(* Logix 5000 AddOnInstructionDefinition export Banner_T30RKD_Param_v4; software revision 33.00 *)

TYPE Banner_IOL_Port_v4 :   // UDT that has all of the data items necessary to communicate with a specific Port on a IO-Link Master
STRUCT
   Port_Controlled : INT;   // Each bit represents a port on an IO-Link Master. Set to 1 to tell AOI to control that port.
   Port_Activate : INT;   // Each bit represents a port on an IO-Link Master. When ON that port will process any commands in queue.
   Port_Read : INT;   // Each bit represents a port on an IO-Link Master. Used to determine when device AOI has requested a Read command.
   Port_Write : INT;   // Each bit represents a port on an IO-Link Master. Used to determine when device AOI has requested a Write command.
   Port_RW_Complete : INT;   // Each bit represents a port on an IO-Link Master. Tells device AOI that Read or Write request has been completed.
   Port_Device_Read : INT;
   Data_Transfer : SINT[190];   // Array to transfer data from IO-Master to device AOIs.
END_STRUCT
END_TYPE

TYPE Banner_T30RKD_RD_v4 :   // UDT that stores the Read Data for a T30RKD.
STRUCT
   Master_Cycle_Time : INT;
   Min_Cycle_Time : INT;
   M_Sequence_Capability : INT;
   IO_Link_Version_ID : INT;
   Process_Data_Input_Length : INT;
   Process_Data_Output_Length : INT;
   Combined_Vendor_ID : DINT;   // IO-Link Vendor ID
   Vendor_ID1 : INT;
   Vendor_ID2 : INT;
   Combined_Device_ID : DINT;   // IO-Link Device ID
   Device_ID1 : INT;
   Device_ID2 : INT;
   Device_ID3 : INT;
   Serial_Number : STRING;
   Teach_State : SINT;   // 0 = Idle, 1 = SP1 Success, 2 = SP2 Success, 3 = SP1 SP2 Success, 4 = Wait for command, 5 = Busy, 7 = Error
   SP1_TP1 : SINT;
   SP1_TP2 : SINT;
   SP2_TP1 : SINT;
   SP2_TP2 : SINT;
   Distance_Meaurement : DINT;
   Excess_Gain : DINT;   // Amount of singal measured over the minimum threshold.
   Stability : SINT;   // 0 = No target, 1 = Marginal target, 2 = Strong target.
   Fault_Status : SINT;   // 0 = No Fault, 1 = Fault Present
   Temperature : DINT;   // Internal Temperature.
   Last_Taught_Temperature : DINT;   // Internal Temperature the last time device was taught.
   All_Time_Run_Time : DINT;   // Read only counter that tracks the total time sensor has been running since manufacture. Value in Hours.
   MDC_Lower_Limit : DINT;
   MDC_Upper_Limit : DINT;
   MDC_Unit : INT;
   MDC_Scale : SINT;
END_STRUCT
END_TYPE

TYPE Banner_T30RKD_v4 :   // All of the parameters for a T30RKD.
STRUCT
   Initial_Global_Read : BOOL;   // Determines if all of the IO-Link data has been read into the PLC yet
   Command : INT;   // Value placed in here will activate a read or write to a specifc IO-Link Index
   Read_Data : Banner_T30RKD_RD_v4;   // Read Only Data
   Write_Data : Banner_T30RKD_WD_v4;   // Write Data
   Archive : Banner_T30RKD_WD_v4;   // Archive Data
   Reset : BOOL;   // Resets AOI. This will force a complete parameter read of the sensor.
END_STRUCT
END_TYPE

TYPE Banner_T30RKD_WD_v4 :   // UDT that stores the Write Data for a T30RKD.
STRUCT
   System_Command : INT;   // See IODD file for list of commands that can be activated via the System Command interface
   Parameter_Access_Lock : SINT;   // Write access to all parameters is prohibited while value is 1. Only this parameter can be adjusted when value is 1.
   Data_Storage_Lock : SINT;   // Automatic data storage is disabled when this value is equal to 1. Read access is not affected.
   Local_Parameterization_Lock : SINT;   // Parameterization via local control elements on device is disabled.
   Local_User_Interface_Lock : SINT;   // Operation of local user interface is disabled.
   Function_Tag : STRING;
   Location_Tag : STRING;
   Teach_in_Channel : SINT;   // 0 = Default, 1 = BDC1, 2 = BDC2
   BDC1_Setpoint_1 : DINT;   // 0 to 15000. SP1 switch point in Switch or Window mode.
   BDC1_Setpoint_2 : DINT;   // 0 to 15000. SP2 switch point in Window mode only.
   BDC1_Switchpoint_Logic : INT;   // 0 = Light Operate, 1 = Dark Operate
   BDC1_Mode : SINT;   // 1 = Switch Mode/Single Mode, 2 = Window Mode
   BDC1_Hysteresis : INT;   // 0 to 15000
   BDC2_Setpoint_1 : DINT;   // 0 to 15000. SP1 switch point in Switch or Window mode.
   BDC2_Setpoint_2 : DINT;   // 0 to 15000. SP2 switch point in Window mode only.
   BDC2_Switchpoint_Logic : INT;   // 0 = Light Operate, 1 = Dark Operate
   BDC2_Mode : SINT;   // 1 = Switch Mode/Single Mode, 2 = Window Mode
   BDC2_Hysteresis : INT;   // 0 to 15000
   Response_Speed : SINT;   // 0 = Fast, 1 = Medium, 2 = Slow
   Peak_Select_Mode : SINT;   // 0 = Strongest Peak, 1 = First Peak
   Sensor_Lockout : SINT;   // 0 = Unlocked, 1 = Locked
   Output_Polarity : SINT;   // 0 = NPN, 1 = PNP
   Process_Data_Filter_Time : INT;   // Time in ms to average process data between updates.
   Process_Data_Layout : SINT;   // 0 = Digital Measurement Sensor, 1 = Distance and Excess Gain, 2 = Distance and Excess Gain with Binary
   Remote_Input_Mode : SINT;   // 0 = Disabled, 1 = Teach
   Amplitude_Threshold : DINT;   // 100 to 5000
   Limit_Filter_Enabled : SINT;   // 0 = Disabled, 1 = Enabled. Rate of change filter for the distance meansurement.
   Limit_Filter_Hold_Time : DINT;   // 50 to 60000. Hold time for when distance change exceeds configured window.
   Limit_Filter_Positive_Distance : DINT;   // 0 to 1000. Window size for distance changes going away from sensor (set 0 to disable)
   Limit_Filter_Negative_Distance : DINT;   // 0 to 1000. Window size for distance changes going towards sensor (set 0 to disable)
   Secondary_Output_Mode : SINT;   // 0 = Independent Output, 1 = Complementary Output, 2 = Pulse Frequency Output
   BDC1_Delay_Timer_1 : DINT;   // 0 to 60000 ms.
   BDC1_Delay_Timer_2 : DINT;   // 0 to 60000 ms
   BDC1_Teach_Offset : DINT;   // -15000 to 15000. Offset applied to taught switch point during single point teach.
   BDC2_Delay_Timer_1 : DINT;   // 0 to 60000 ms
   BDC2_Delay_Timer_2 : DINT;   // 0 to 60000 ms
   BDC2_Teach_Offset : DINT;   // -15000 to 15000. Offset applied to taught switch point during single point teach.
   Resettable_Run_Time : DINT;
   Loss_of_Signal : SINT;   // 0 = Hold, 1 = Low, 2 = High
   SP1_PFM_Setpoint : DINT;   // 0 to 15000 in Hz
   SP2_PFM_Setpoint : DINT;   // 0 to 15000 in Hz
   All_Time_Run_Time_Event_Time : DINT;
   Resettable_Run_Time_Event_Time : DINT;
   Active_Sensing_Range_Near : DINT;   // 0 to 16000. Near measurement limit of sensing range.
   Active_Sensing_Range_Far : DINT;   // 0 to 16000. Far measurement limit of sensing range.
END_STRUCT
END_TYPE

ADD_ON_INSTRUCTION Banner_T30RKD_Param_v4   (* revision 4.0, vendor Banner Engineering *)
// AOI to read and write parameter data to an IO-Link T30R Dual Discrete.
VAR_IN_OUT
   T30RKD : Banner_T30RKD_v4; {required}
   Port_Data : Banner_IOL_Port_v4; {required}
END_VAR
VAR_INPUT
   Port : DINT; {required}
END_VAR
VAR
   Local_Control : DINT; {access None}
   Global_Read_Command_Value : INT; {access None}
   Global_Write_Command_Value : INT; {access None}
   Command_Being_Processed : BOOL; {access None}
   Update_Archive : BOOL; {access None}
   Index_Write_Inprocess : DINT; {access None}
   Index_Write_Control : DINT; {access None}
   Inprocess_Index : DINT; {access None}
END_VAR

ROUTINE Logic   (* ladder *)
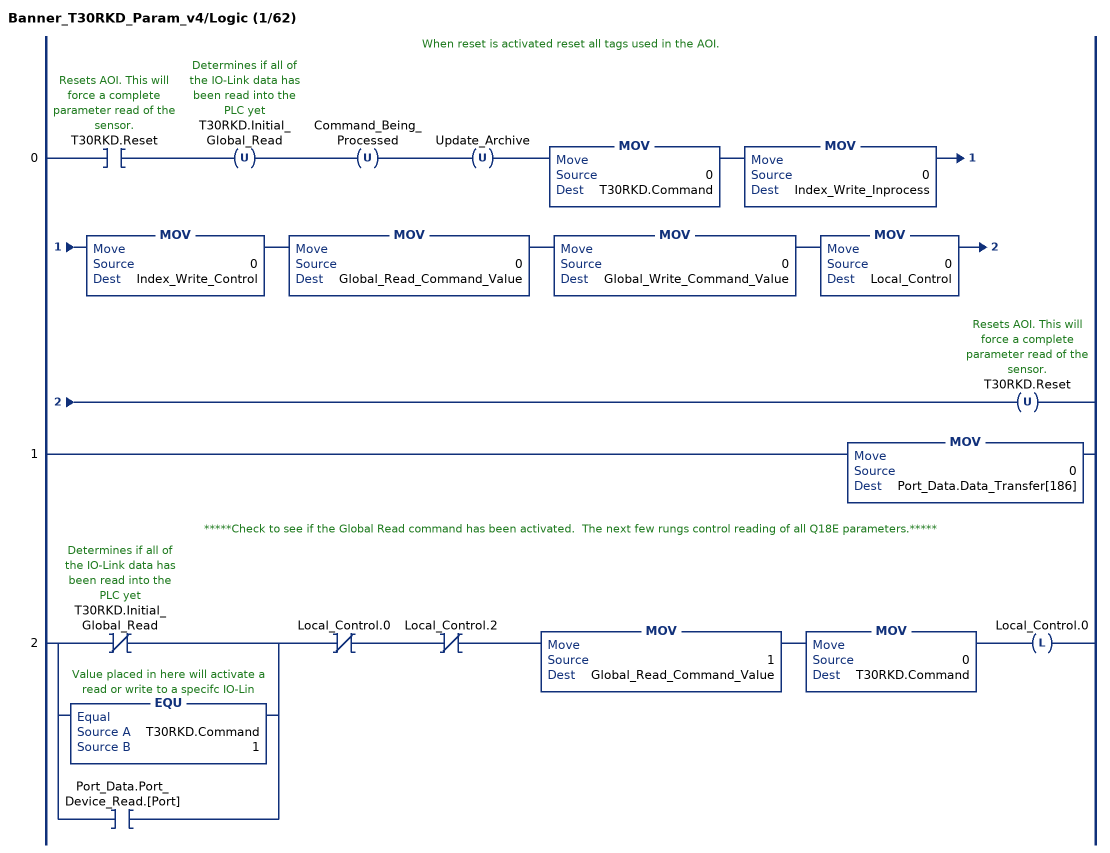
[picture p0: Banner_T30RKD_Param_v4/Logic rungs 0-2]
   // When reset is activated reset all tags used in the AOI.
   0: XIC(T30RKD.Reset)OTU(T30RKD.Initial_Global_Read)OTU(Command_Being_Processed)OTU(Update_Archive)MOV(0,T30RKD.Command)MOV(0,Index_Write_Inprocess)MOV(0,Index_Write_Control)MOV(0,Global_Read_Command_Value)MOV(0,Global_Write_Command_Value)MOV(0,Local_Control)OTU(T30RKD.Reset);
   1: MOV(0,Port_Data.Data_Transfer[186]);
   // *****Check to see if the Global Read command has been activated.  The next few rungs control reading of all Q18E parameters.*****
   2: [XIO(T30RKD.Initial_Global_Read) ,EQU(T30RKD.Command,1) ,XIC(Port_Data.Port_Device_Read.[Port]) ]XIO(Local_Control.0)XIO(Local_Control.2)MOV(1,Global_Read_Command_Value)MOV(0,T30RKD.Command)OTL(Local_Control.0);
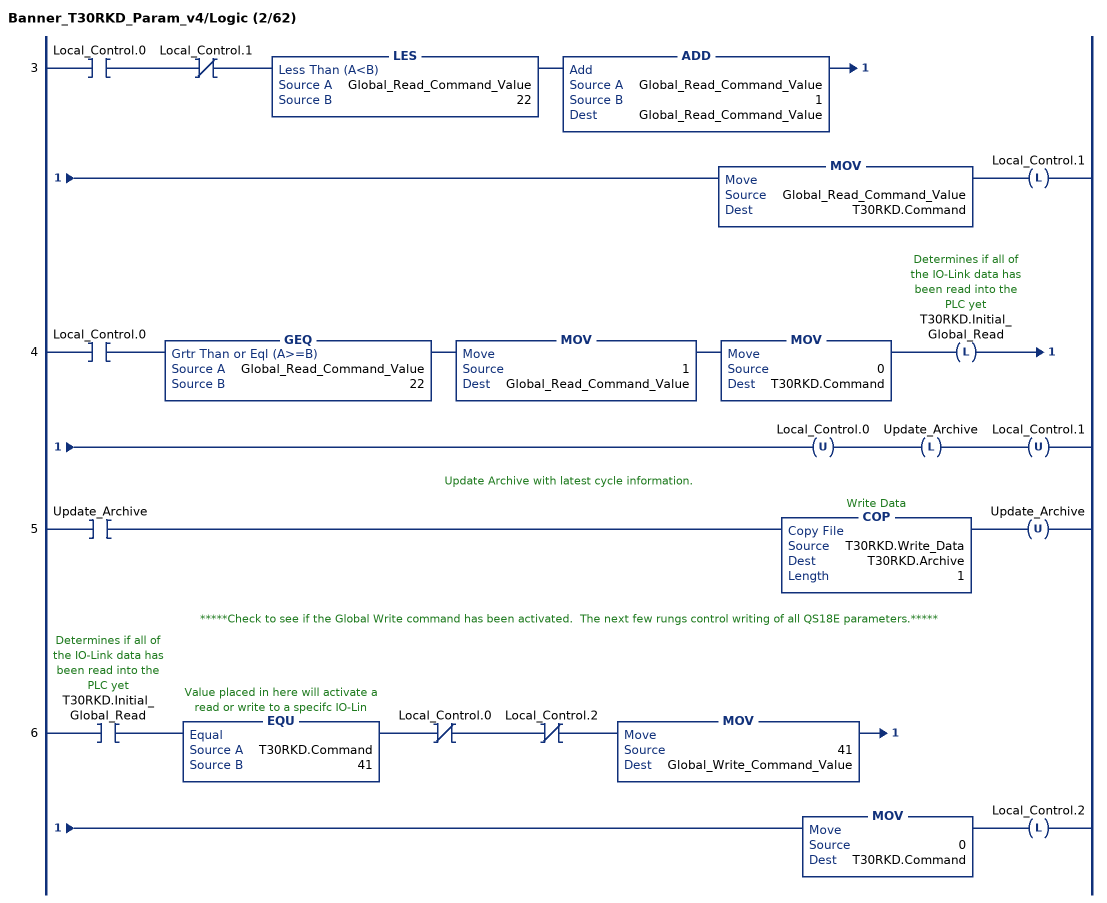
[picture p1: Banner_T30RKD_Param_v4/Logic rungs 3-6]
   3: XIC(Local_Control.0)XIO(Local_Control.1)LES(Global_Read_Command_Value,22)ADD(Global_Read_Command_Value,1,Global_Read_Command_Value)MOV(Global_Read_Command_Value,T30RKD.Command)OTL(Local_Control.1);
   4: XIC(Local_Control.0)GEQ(Global_Read_Command_Value,22)MOV(1,Global_Read_Command_Value)MOV(0,T30RKD.Command)OTL(T30RKD.Initial_Global_Read)OTU(Local_Control.0)OTL(Update_Archive)OTU(Local_Control.1);
   // Update Archive with latest cycle information.
   5: XIC(Update_Archive)COP(T30RKD.Write_Data,T30RKD.Archive,1)OTU(Update_Archive);
   // *****Check to see if the Global Write command has been activated.  The next few rungs control writing of all QS18E parameters.*****
   6: XIC(T30RKD.Initial_Global_Read)EQU(T30RKD.Command,41)XIO(Local_Control.0)XIO(Local_Control.2)MOV(41,Global_Write_Command_Value)MOV(0,T30RKD.Command)OTL(Local_Control.2);
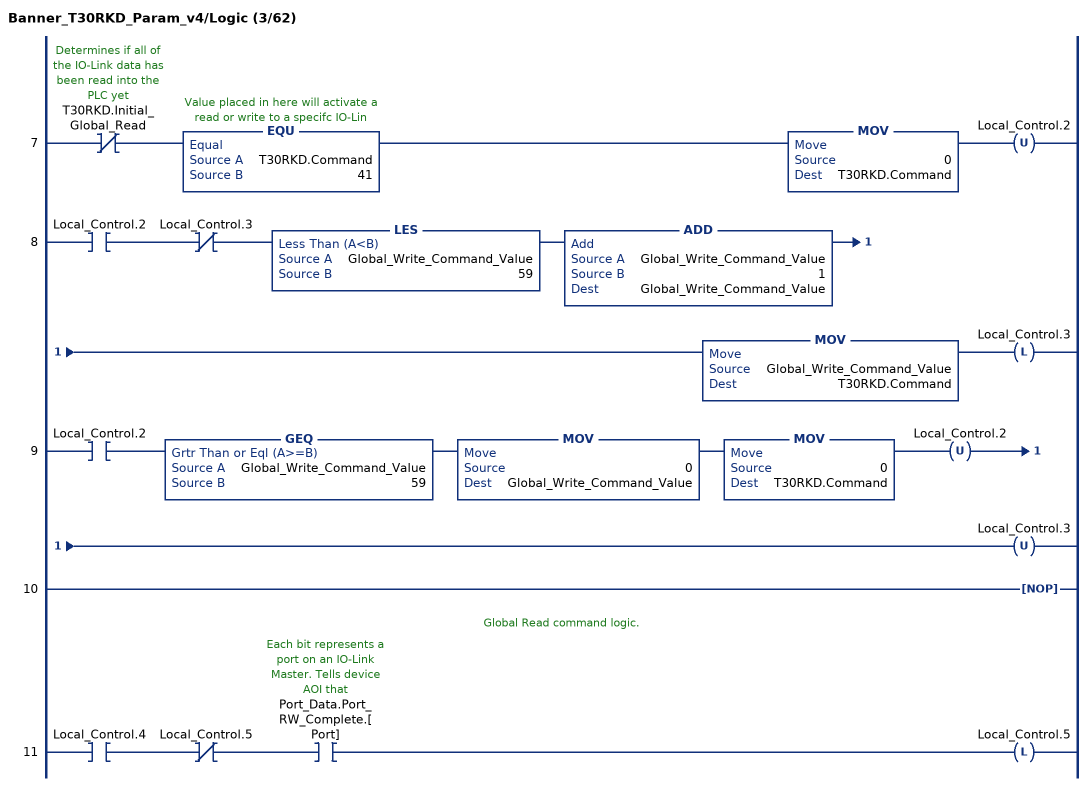
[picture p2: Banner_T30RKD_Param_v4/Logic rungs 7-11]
   7: XIO(T30RKD.Initial_Global_Read)EQU(T30RKD.Command,41)MOV(0,T30RKD.Command)OTU(Local_Control.2);
   8: XIC(Local_Control.2)XIO(Local_Control.3)LES(Global_Write_Command_Value,59)ADD(Global_Write_Command_Value,1,Global_Write_Command_Value)MOV(Global_Write_Command_Value,T30RKD.Command)OTL(Local_Control.3);
   9: XIC(Local_Control.2)GEQ(Global_Write_Command_Value,59)MOV(0,Global_Write_Command_Value)MOV(0,T30RKD.Command)OTU(Local_Control.2)OTU(Local_Control.3);
   10: NOP();
   // Global Read command logic.
   11: XIC(Local_Control.4)XIO(Local_Control.5)XIC(Port_Data.Port_RW_Complete.[Port])OTL(Local_Control.5);
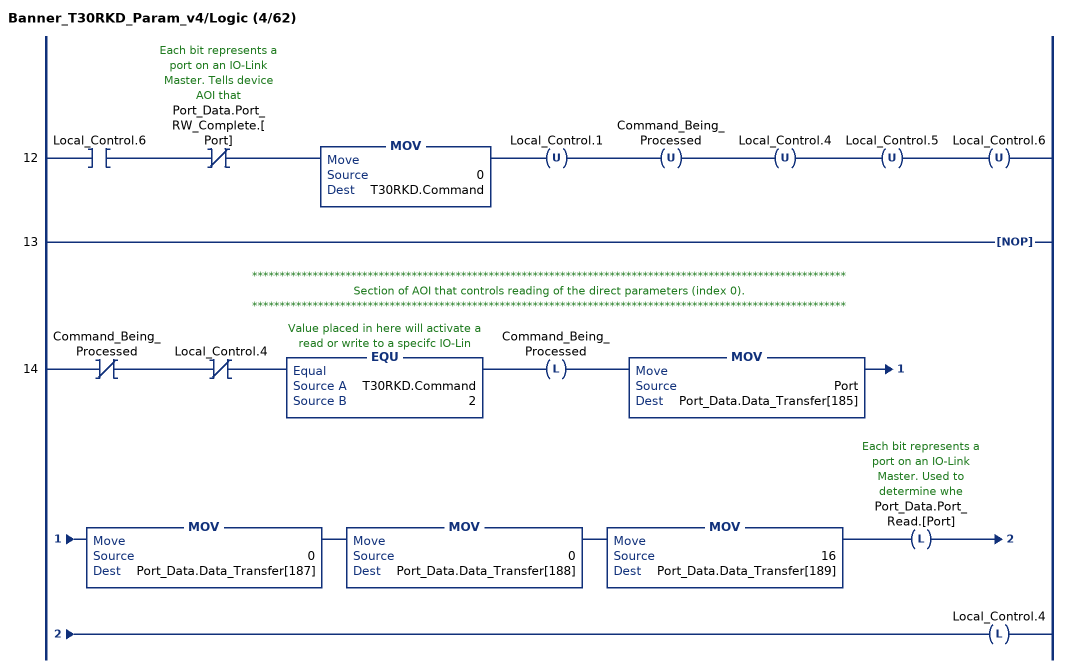
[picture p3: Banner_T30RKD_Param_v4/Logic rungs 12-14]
   12: XIC(Local_Control.6)XIO(Port_Data.Port_RW_Complete.[Port])MOV(0,T30RKD.Command)OTU(Local_Control.1)OTU(Command_Being_Processed)OTU(Local_Control.4)OTU(Local_Control.5)OTU(Local_Control.6);
   13: NOP();
   // ************************************************************************************************************
   // Section of AOI that controls reading of the direct parameters (index 0).
   // ************************************************************************************************************
   14: XIO(Command_Being_Processed)XIO(Local_Control.4)EQU(T30RKD.Command,2)OTL(Command_Being_Processed)MOV(Port,Port_Data.Data_Transfer[185])MOV(0,Port_Data.Data_Transfer[187])MOV(0,Port_Data.Data_Transfer[188])MOV(16,Port_Data.Data_Transfer[189])OTL(Port_Data.Port_Read.[Port])OTL(Local_Control.4);
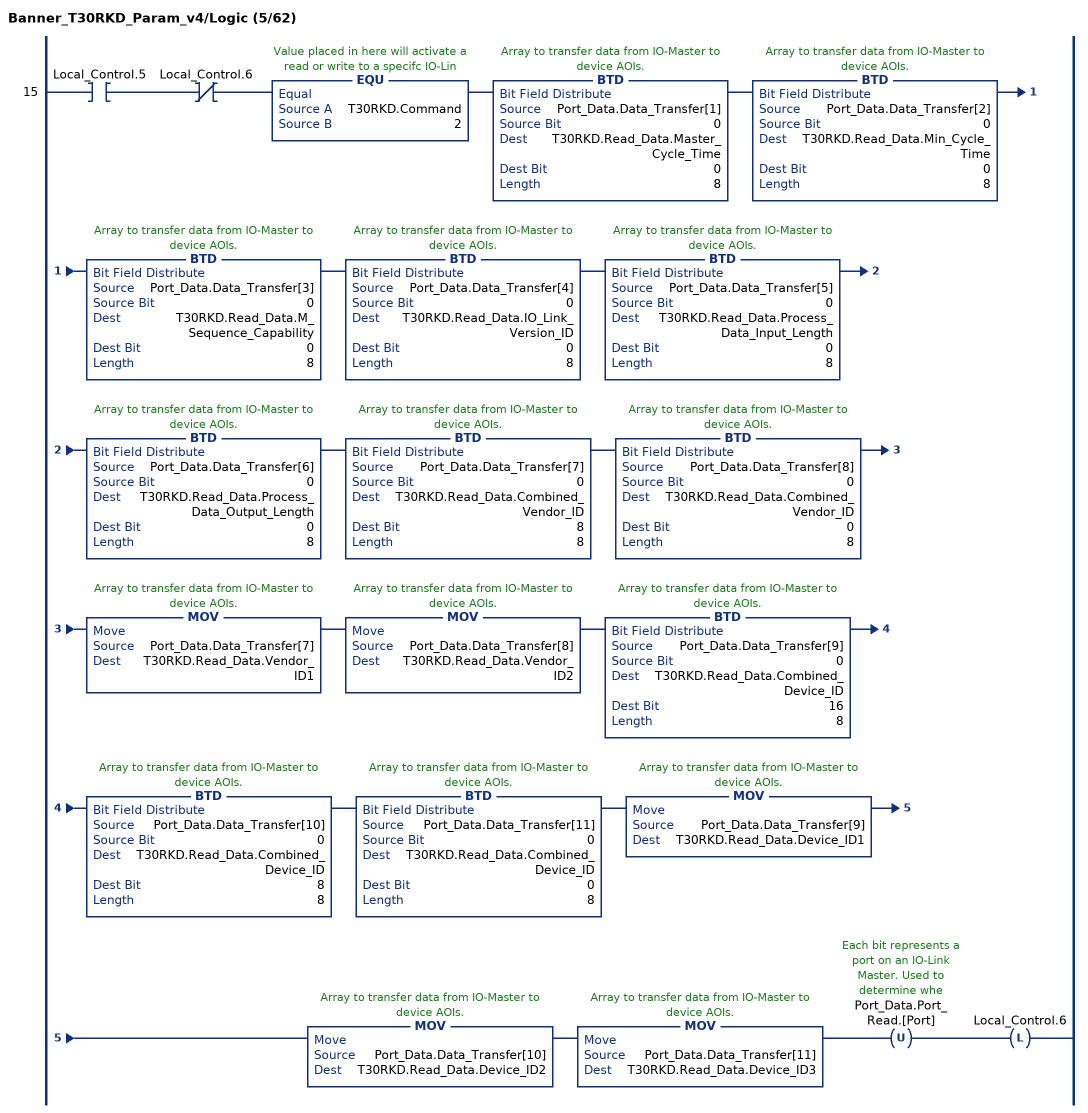
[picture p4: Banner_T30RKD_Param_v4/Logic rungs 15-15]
   15: XIC(Local_Control.5)XIO(Local_Control.6)EQU(T30RKD.Command,2)BTD(Port_Data.Data_Transfer[1],0,T30RKD.Read_Data.Master_Cycle_Time,0,8)BTD(Port_Data.Data_Transfer[2],0,T30RKD.Read_Data.Min_Cycle_Time,0,8)BTD(Port_Data.Data_Transfer[3],0,T30RKD.Read_Data.M_Sequence_Capability,0,8)BTD(Port_Data.Data_Transfer[4],0,T30RKD.Read_Data.IO_Link_Version_ID,0,8)BTD(Port_Data.Data_Transfer[5],0,T30RKD.Read_Data.Process_Data_Input_Length,0,8)BTD(Port_Data.Data_Transfer[6],0,T30RKD.Read_Data.Process_Data_Output_Length,0,8)BTD(Port_Data.Data_Transfer[7],0,T30RKD.Read_Data.Combined_Vendor_ID,8,8)BTD(Port_Data.Data_Transfer[8],0,T30RKD.Read_Data.Combined_Vendor_ID,0,8)MOV(Port_Data.Data_Transfer[7],T30RKD.Read_Data.Vendor_ID1)MOV(Port_Data.Data_Transfer[8],T30RKD.Read_Data.Vendor_ID2)BTD(Port_Data.Data_Transfer[9],0,T30RKD.Read_Data.Combined_Device_ID,16,8)BTD(Port_Data.Data_Transfer[10],0,T30RKD.Read_Data.Combined_Device_ID,8,8)BTD(Port_Data.Data_Transfer[11],0,T30RKD.Read_Data.Combined_Device_ID,0,8)MOV(Port_Data.Data_Transfer[9],T30RKD.Read_Data.Device_ID1)MOV(Port_Data.Data_Transfer[10],T30RKD.Read_Data.Device_ID2)MOV(Port_Data.Data_Transfer[11],T30RKD.Read_Data.Device_ID3)OTU(Port_Data.Port_Read.[Port])OTL(Local_Control.6);
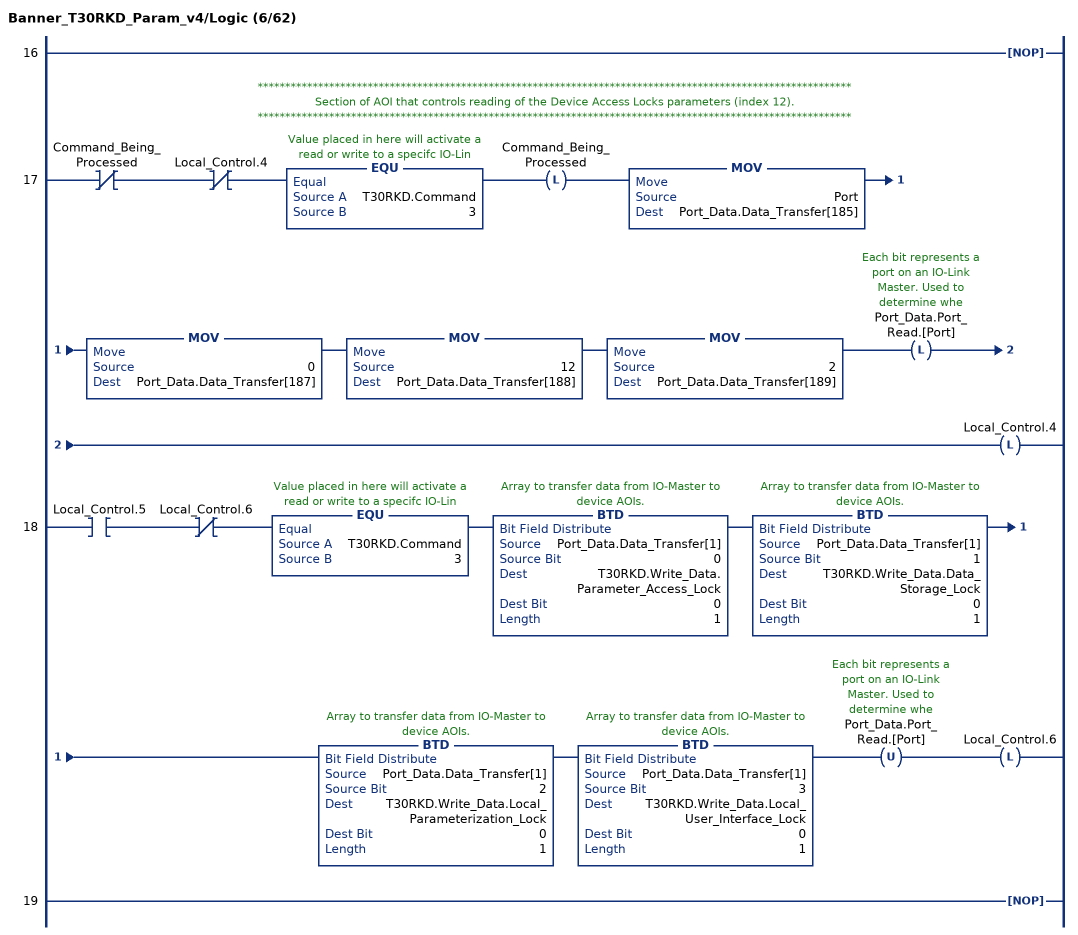
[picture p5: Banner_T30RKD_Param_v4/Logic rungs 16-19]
   16: NOP();
   // ************************************************************************************************************
   // Section of AOI that controls reading of the Device Access Locks parameters (index 12).
   // ************************************************************************************************************
   17: XIO(Command_Being_Processed)XIO(Local_Control.4)EQU(T30RKD.Command,3)OTL(Command_Being_Processed)MOV(Port,Port_Data.Data_Transfer[185])MOV(0,Port_Data.Data_Transfer[187])MOV(12,Port_Data.Data_Transfer[188])MOV(2,Port_Data.Data_Transfer[189])OTL(Port_Data.Port_Read.[Port])OTL(Local_Control.4);
   18: XIC(Local_Control.5)XIO(Local_Control.6)EQU(T30RKD.Command,3)BTD(Port_Data.Data_Transfer[1],0,T30RKD.Write_Data.Parameter_Access_Lock,0,1)BTD(Port_Data.Data_Transfer[1],1,T30RKD.Write_Data.Data_Storage_Lock,0,1)BTD(Port_Data.Data_Transfer[1],2,T30RKD.Write_Data.Local_Parameterization_Lock,0,1)BTD(Port_Data.Data_Transfer[1],3,T30RKD.Write_Data.Local_User_Interface_Lock,0,1)OTU(Port_Data.Port_Read.[Port])OTL(Local_Control.6);
   19: NOP();
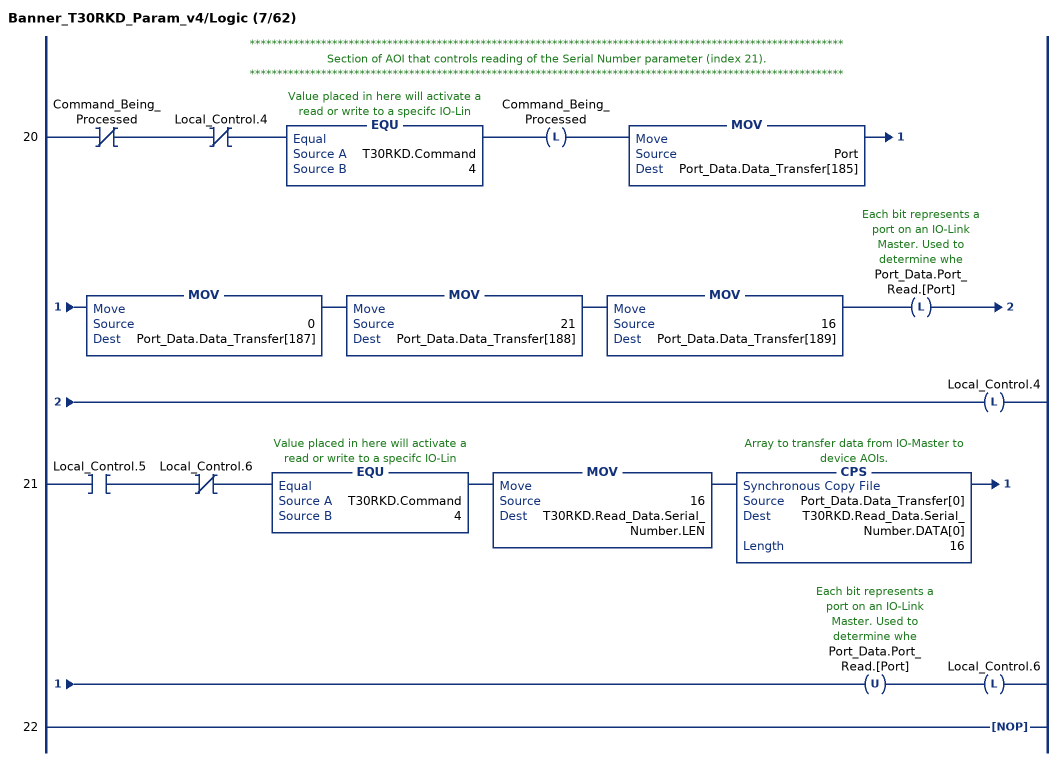
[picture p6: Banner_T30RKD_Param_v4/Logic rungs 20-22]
   // ************************************************************************************************************
   // Section of AOI that controls reading of the Serial Number parameter (index 21).
   // ************************************************************************************************************
   20: XIO(Command_Being_Processed)XIO(Local_Control.4)EQU(T30RKD.Command,4)OTL(Command_Being_Processed)MOV(Port,Port_Data.Data_Transfer[185])MOV(0,Port_Data.Data_Transfer[187])MOV(21,Port_Data.Data_Transfer[188])MOV(16,Port_Data.Data_Transfer[189])OTL(Port_Data.Port_Read.[Port])OTL(Local_Control.4);
   21: XIC(Local_Control.5)XIO(Local_Control.6)EQU(T30RKD.Command,4)MOV(16,T30RKD.Read_Data.Serial_Number.LEN)CPS(Port_Data.Data_Transfer[0],T30RKD.Read_Data.Serial_Number.DATA[0],16)OTU(Port_Data.Port_Read.[Port])OTL(Local_Control.6);
   22: NOP();
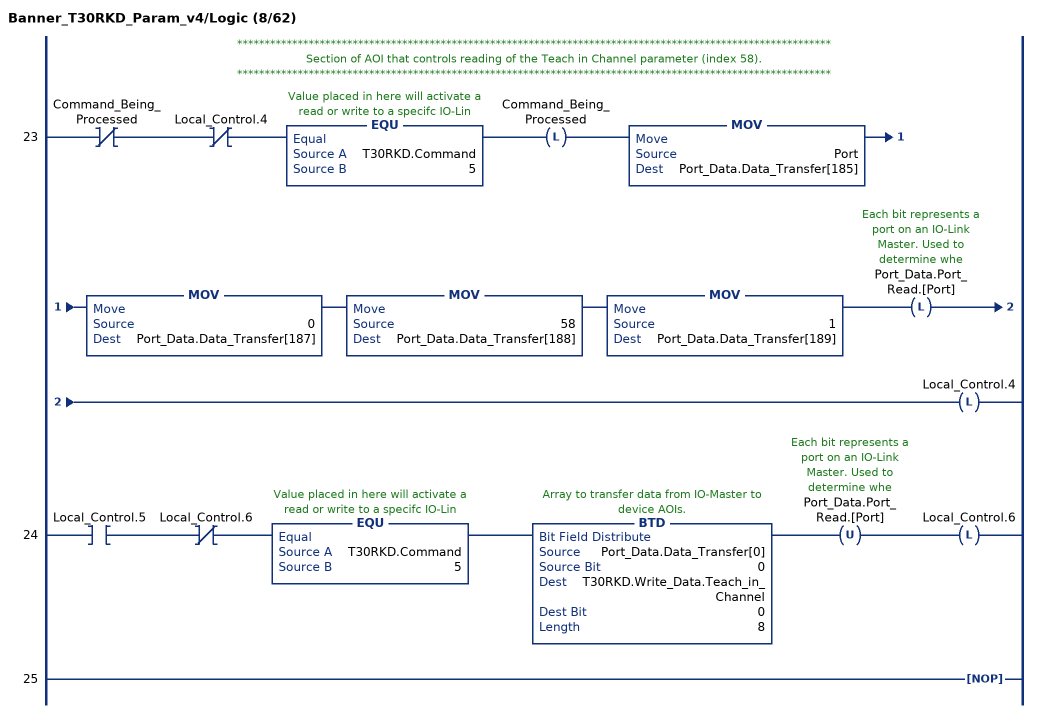
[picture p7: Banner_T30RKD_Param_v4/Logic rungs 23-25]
   // ************************************************************************************************************
   // Section of AOI that controls reading of the Teach in Channel parameter (index 58).
   // ************************************************************************************************************
   23: XIO(Command_Being_Processed)XIO(Local_Control.4)EQU(T30RKD.Command,5)OTL(Command_Being_Processed)MOV(Port,Port_Data.Data_Transfer[185])MOV(0,Port_Data.Data_Transfer[187])MOV(58,Port_Data.Data_Transfer[188])MOV(1,Port_Data.Data_Transfer[189])OTL(Port_Data.Port_Read.[Port])OTL(Local_Control.4);
   24: XIC(Local_Control.5)XIO(Local_Control.6)EQU(T30RKD.Command,5)BTD(Port_Data.Data_Transfer[0],0,T30RKD.Write_Data.Teach_in_Channel,0,8)OTU(Port_Data.Port_Read.[Port])OTL(Local_Control.6);
   25: NOP();
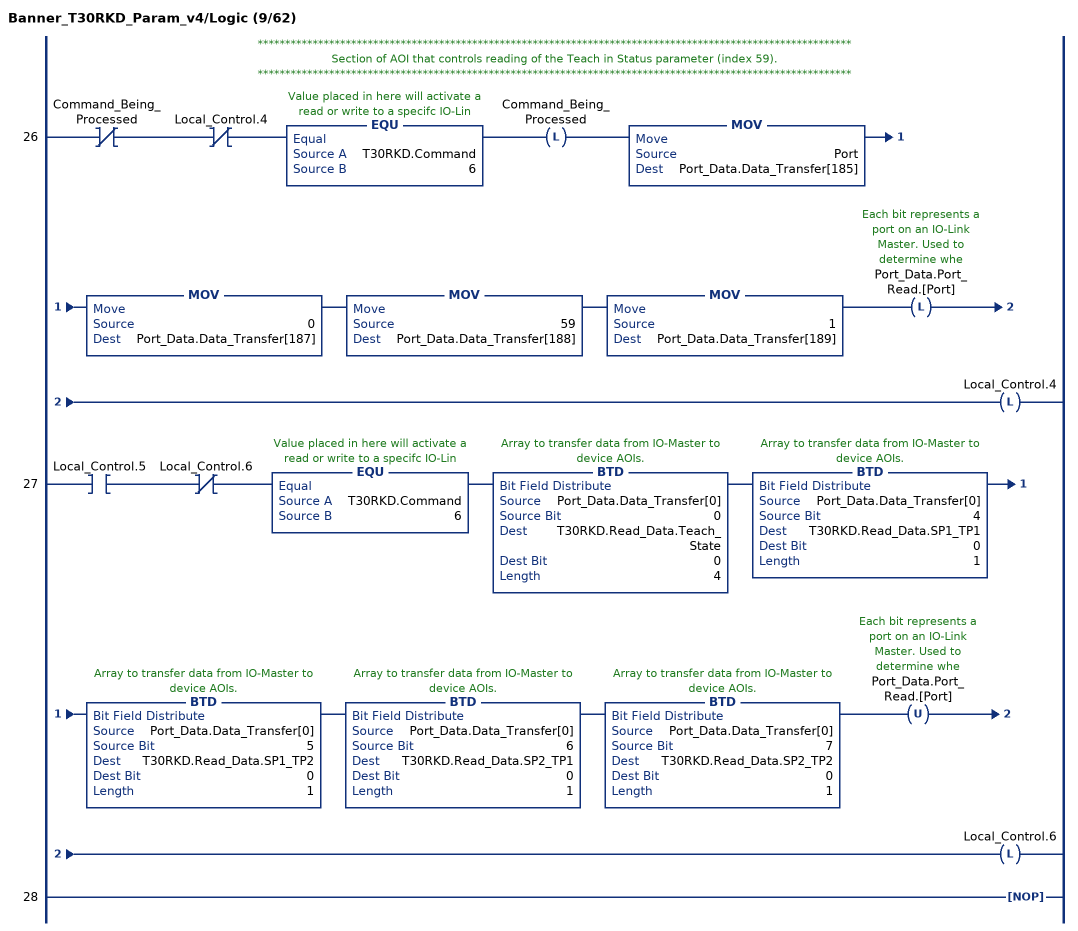
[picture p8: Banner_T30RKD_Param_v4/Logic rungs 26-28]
   // ************************************************************************************************************
   // Section of AOI that controls reading of the Teach in Status parameter (index 59).
   // ************************************************************************************************************
   26: XIO(Command_Being_Processed)XIO(Local_Control.4)EQU(T30RKD.Command,6)OTL(Command_Being_Processed)MOV(Port,Port_Data.Data_Transfer[185])MOV(0,Port_Data.Data_Transfer[187])MOV(59,Port_Data.Data_Transfer[188])MOV(1,Port_Data.Data_Transfer[189])OTL(Port_Data.Port_Read.[Port])OTL(Local_Control.4);
   27: XIC(Local_Control.5)XIO(Local_Control.6)EQU(T30RKD.Command,6)BTD(Port_Data.Data_Transfer[0],0,T30RKD.Read_Data.Teach_State,0,4)BTD(Port_Data.Data_Transfer[0],4,T30RKD.Read_Data.SP1_TP1,0,1)BTD(Port_Data.Data_Transfer[0],5,T30RKD.Read_Data.SP1_TP2,0,1)BTD(Port_Data.Data_Transfer[0],6,T30RKD.Read_Data.SP2_TP1,0,1)BTD(Port_Data.Data_Transfer[0],7,T30RKD.Read_Data.SP2_TP2,0,1)OTU(Port_Data.Port_Read.[Port])OTL(Local_Control.6);
   28: NOP();
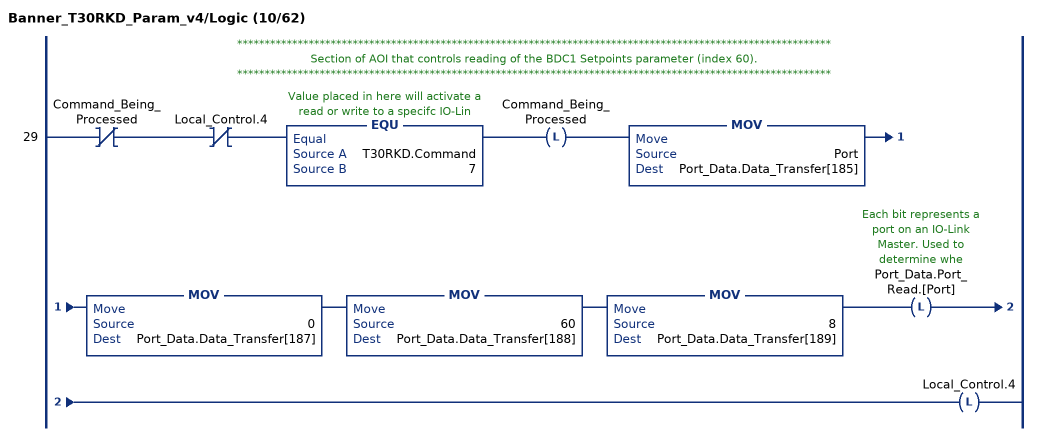
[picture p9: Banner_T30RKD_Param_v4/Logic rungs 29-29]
   // ************************************************************************************************************
   // Section of AOI that controls reading of the BDC1 Setpoints parameter (index 60).
   // ************************************************************************************************************
   29: XIO(Command_Being_Processed)XIO(Local_Control.4)EQU(T30RKD.Command,7)OTL(Command_Being_Processed)MOV(Port,Port_Data.Data_Transfer[185])MOV(0,Port_Data.Data_Transfer[187])MOV(60,Port_Data.Data_Transfer[188])MOV(8,Port_Data.Data_Transfer[189])OTL(Port_Data.Port_Read.[Port])OTL(Local_Control.4);
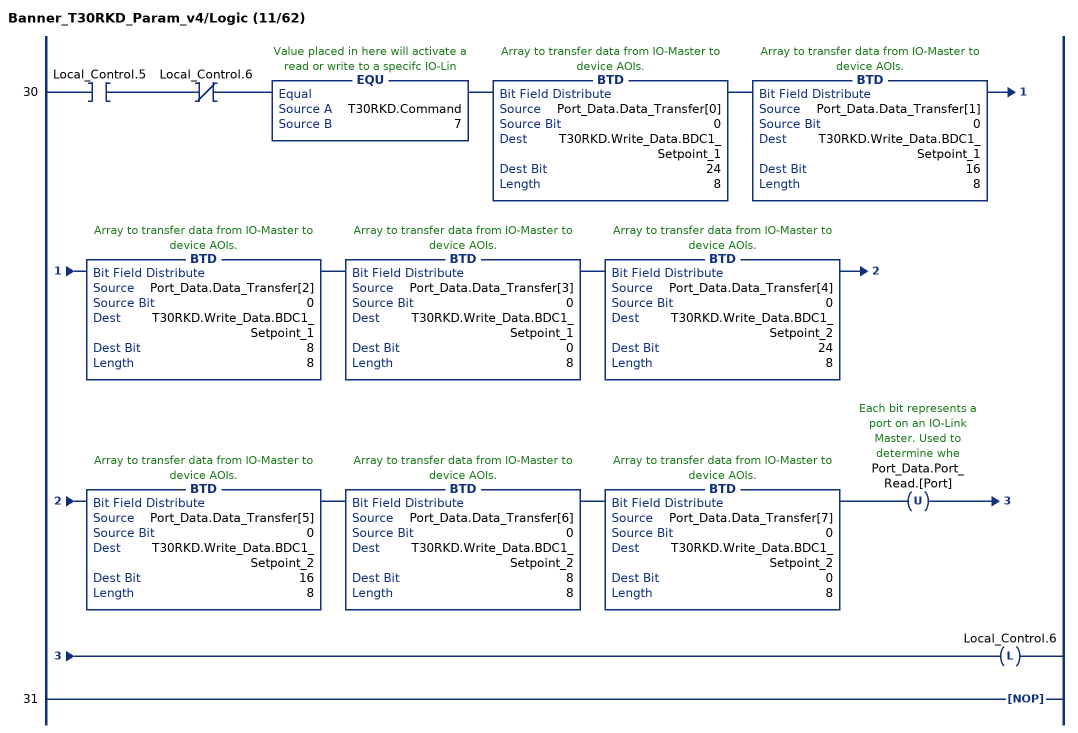
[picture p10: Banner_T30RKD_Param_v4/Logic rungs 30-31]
   30: XIC(Local_Control.5)XIO(Local_Control.6)EQU(T30RKD.Command,7)BTD(Port_Data.Data_Transfer[0],0,T30RKD.Write_Data.BDC1_Setpoint_1,24,8)BTD(Port_Data.Data_Transfer[1],0,T30RKD.Write_Data.BDC1_Setpoint_1,16,8)BTD(Port_Data.Data_Transfer[2],0,T30RKD.Write_Data.BDC1_Setpoint_1,8,8)BTD(Port_Data.Data_Transfer[3],0,T30RKD.Write_Data.BDC1_Setpoint_1,0,8)BTD(Port_Data.Data_Transfer[4],0,T30RKD.Write_Data.BDC1_Setpoint_2,24,8)BTD(Port_Data.Data_Transfer[5],0,T30RKD.Write_Data.BDC1_Setpoint_2,16,8)BTD(Port_Data.Data_Transfer[6],0,T30RKD.Write_Data.BDC1_Setpoint_2,8,8)BTD(Port_Data.Data_Transfer[7],0,T30RKD.Write_Data.BDC1_Setpoint_2,0,8)OTU(Port_Data.Port_Read.[Port])OTL(Local_Control.6);
   31: NOP();
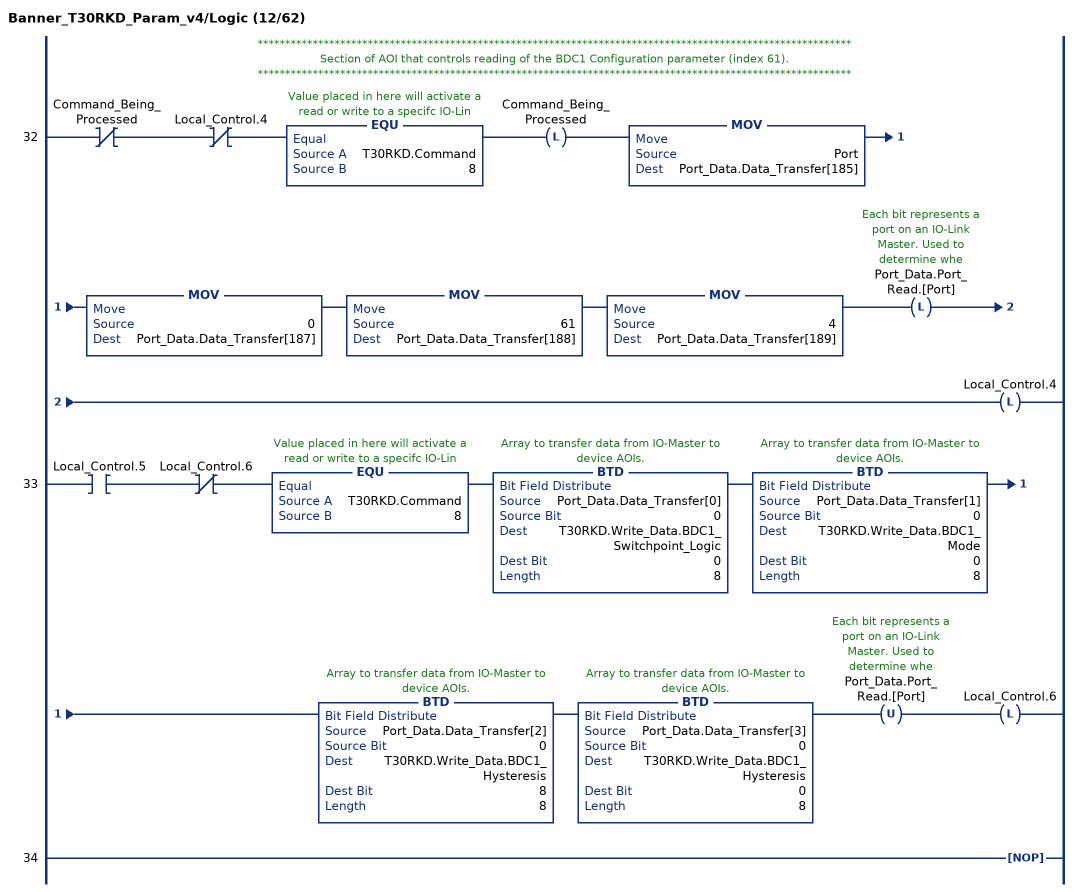
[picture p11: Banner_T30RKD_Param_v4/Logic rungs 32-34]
   // ************************************************************************************************************
   // Section of AOI that controls reading of the BDC1 Configuration parameter (index 61).
   // ************************************************************************************************************
   32: XIO(Command_Being_Processed)XIO(Local_Control.4)EQU(T30RKD.Command,8)OTL(Command_Being_Processed)MOV(Port,Port_Data.Data_Transfer[185])MOV(0,Port_Data.Data_Transfer[187])MOV(61,Port_Data.Data_Transfer[188])MOV(4,Port_Data.Data_Transfer[189])OTL(Port_Data.Port_Read.[Port])OTL(Local_Control.4);
   33: XIC(Local_Control.5)XIO(Local_Control.6)EQU(T30RKD.Command,8)BTD(Port_Data.Data_Transfer[0],0,T30RKD.Write_Data.BDC1_Switchpoint_Logic,0,8)BTD(Port_Data.Data_Transfer[1],0,T30RKD.Write_Data.BDC1_Mode,0,8)BTD(Port_Data.Data_Transfer[2],0,T30RKD.Write_Data.BDC1_Hysteresis,8,8)BTD(Port_Data.Data_Transfer[3],0,T30RKD.Write_Data.BDC1_Hysteresis,0,8)OTU(Port_Data.Port_Read.[Port])OTL(Local_Control.6);
   34: NOP();
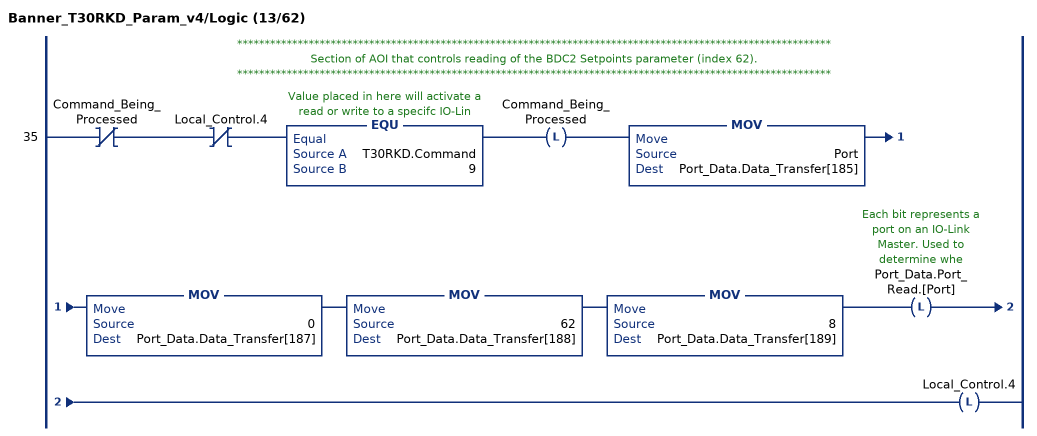
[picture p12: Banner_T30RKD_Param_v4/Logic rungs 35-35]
   // ************************************************************************************************************
   // Section of AOI that controls reading of the BDC2 Setpoints parameter (index 62).
   // ************************************************************************************************************
   35: XIO(Command_Being_Processed)XIO(Local_Control.4)EQU(T30RKD.Command,9)OTL(Command_Being_Processed)MOV(Port,Port_Data.Data_Transfer[185])MOV(0,Port_Data.Data_Transfer[187])MOV(62,Port_Data.Data_Transfer[188])MOV(8,Port_Data.Data_Transfer[189])OTL(Port_Data.Port_Read.[Port])OTL(Local_Control.4);
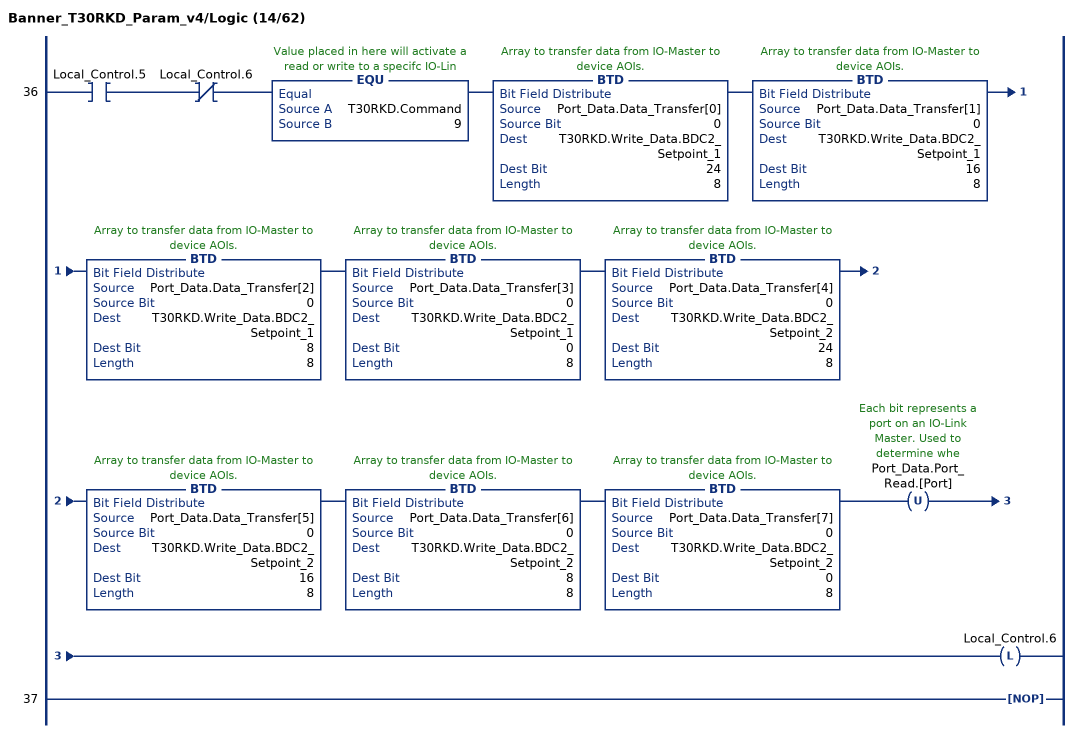
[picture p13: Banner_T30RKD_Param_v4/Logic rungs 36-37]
   36: XIC(Local_Control.5)XIO(Local_Control.6)EQU(T30RKD.Command,9)BTD(Port_Data.Data_Transfer[0],0,T30RKD.Write_Data.BDC2_Setpoint_1,24,8)BTD(Port_Data.Data_Transfer[1],0,T30RKD.Write_Data.BDC2_Setpoint_1,16,8)BTD(Port_Data.Data_Transfer[2],0,T30RKD.Write_Data.BDC2_Setpoint_1,8,8)BTD(Port_Data.Data_Transfer[3],0,T30RKD.Write_Data.BDC2_Setpoint_1,0,8)BTD(Port_Data.Data_Transfer[4],0,T30RKD.Write_Data.BDC2_Setpoint_2,24,8)BTD(Port_Data.Data_Transfer[5],0,T30RKD.Write_Data.BDC2_Setpoint_2,16,8)BTD(Port_Data.Data_Transfer[6],0,T30RKD.Write_Data.BDC2_Setpoint_2,8,8)BTD(Port_Data.Data_Transfer[7],0,T30RKD.Write_Data.BDC2_Setpoint_2,0,8)OTU(Port_Data.Port_Read.[Port])OTL(Local_Control.6);
   37: NOP();
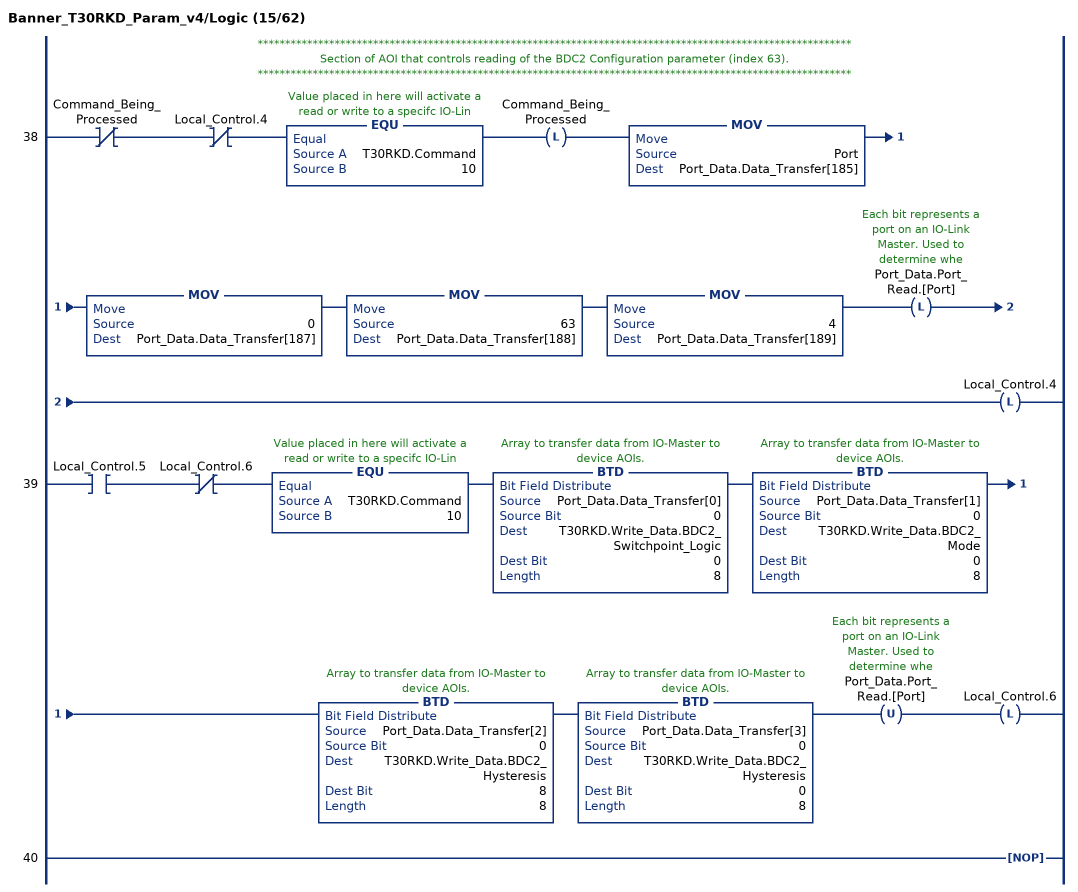
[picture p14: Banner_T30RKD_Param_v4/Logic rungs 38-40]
   // ************************************************************************************************************
   // Section of AOI that controls reading of the BDC2 Configuration parameter (index 63).
   // ************************************************************************************************************
   38: XIO(Command_Being_Processed)XIO(Local_Control.4)EQU(T30RKD.Command,10)OTL(Command_Being_Processed)MOV(Port,Port_Data.Data_Transfer[185])MOV(0,Port_Data.Data_Transfer[187])MOV(63,Port_Data.Data_Transfer[188])MOV(4,Port_Data.Data_Transfer[189])OTL(Port_Data.Port_Read.[Port])OTL(Local_Control.4);
   39: XIC(Local_Control.5)XIO(Local_Control.6)EQU(T30RKD.Command,10)BTD(Port_Data.Data_Transfer[0],0,T30RKD.Write_Data.BDC2_Switchpoint_Logic,0,8)BTD(Port_Data.Data_Transfer[1],0,T30RKD.Write_Data.BDC2_Mode,0,8)BTD(Port_Data.Data_Transfer[2],0,T30RKD.Write_Data.BDC2_Hysteresis,8,8)BTD(Port_Data.Data_Transfer[3],0,T30RKD.Write_Data.BDC2_Hysteresis,0,8)OTU(Port_Data.Port_Read.[Port])OTL(Local_Control.6);
   40: NOP();
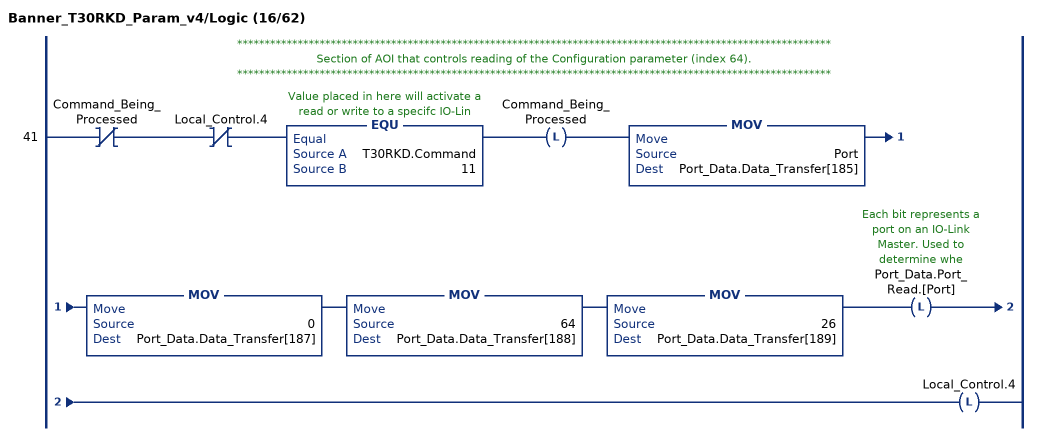
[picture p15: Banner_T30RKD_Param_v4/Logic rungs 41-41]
   // ************************************************************************************************************
   // Section of AOI that controls reading of the Configuration parameter (index 64).
   // ************************************************************************************************************
   41: XIO(Command_Being_Processed)XIO(Local_Control.4)EQU(T30RKD.Command,11)OTL(Command_Being_Processed)MOV(Port,Port_Data.Data_Transfer[185])MOV(0,Port_Data.Data_Transfer[187])MOV(64,Port_Data.Data_Transfer[188])MOV(26,Port_Data.Data_Transfer[189])OTL(Port_Data.Port_Read.[Port])OTL(Local_Control.4);
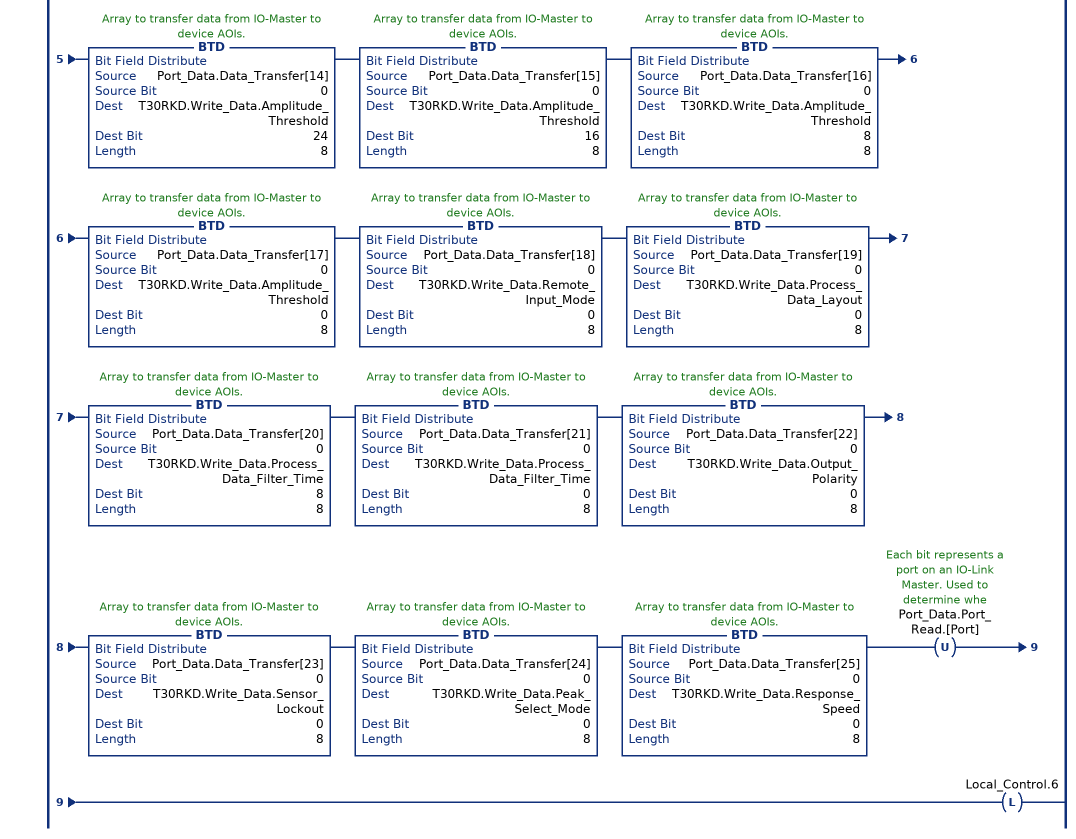
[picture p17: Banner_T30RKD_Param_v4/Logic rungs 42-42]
   42: XIC(Local_Control.5)XIO(Local_Control.6)EQU(T30RKD.Command,11)BTD(Port_Data.Data_Transfer[0],0,T30RKD.Write_Data.Secondary_Output_Mode,0,8)BTD(Port_Data.Data_Transfer[1],0,T30RKD.Write_Data.Limit_Filter_Negative_Distance,24,8)BTD(Port_Data.Data_Transfer[2],0,T30RKD.Write_Data.Limit_Filter_Negative_Distance,16,8)BTD(Port_Data.Data_Transfer[3],0,T30RKD.Write_Data.Limit_Filter_Negative_Distance,8,8)BTD(Port_Data.Data_Transfer[4],0,T30RKD.Write_Data.Limit_Filter_Negative_Distance,0,8)BTD(Port_Data.Data_Transfer[5],0,T30RKD.Write_Data.Limit_Filter_Positive_Distance,24,8)BTD(Port_Data.Data_Transfer[6],0,T30RKD.Write_Data.Limit_Filter_Positive_Distance,16,8)BTD(Port_Data.Data_Transfer[7],0,T30RKD.Write_Data.Limit_Filter_Positive_Distance,8,8)BTD(Port_Data.Data_Transfer[8],0,T30RKD.Write_Data.Limit_Filter_Positive_Distance,0,8)BTD(Port_Data.Data_Transfer[9],0,T30RKD.Write_Data.Limit_Filter_Hold_Time,24,8)BTD(Port_Data.Data_Transfer[10],0,T30RKD.Write_Data.Limit_Filter_Hold_Time,16,8)BTD(Port_Data.Data_Transfer[11],0,T30RKD.Write_Data.Limit_Filter_Hold_Time,8,8)BTD(Port_Data.Data_Transfer[12],0,T30RKD.Write_Data.Limit_Filter_Hold_Time,0,8)BTD(Port_Data.Data_Transfer[13],0,T30RKD.Write_Data.Limit_Filter_Enabled,0,8)BTD(Port_Data.Data_Transfer[14],0,T30RKD.Write_Data.Amplitude_Threshold,24,8)BTD(Port_Data.Data_Transfer[15],0,T30RKD.Write_Data.Amplitude_Threshold,16,8)BTD(Port_Data.Data_Transfer[16],0,T30RKD.Write_Data.Amplitude_Threshold,8,8)BTD(Port_Data.Data_Transfer[17],0,T30RKD.Write_Data.Amplitude_Threshold,0,8)BTD(Port_Data.Data_Transfer[18],0,T30RKD.Write_Data.Remote_Input_Mode,0,8)BTD(Port_Data.Data_Transfer[19],0,T30RKD.Write_Data.Process_Data_Layout,0,8)BTD(Port_Data.Data_Transfer[20],0,T30RKD.Write_Data.Process_Data_Filter_Time,8,8)BTD(Port_Data.Data_Transfer[21],0,T30RKD.Write_Data.Process_Data_Filter_Time,0,8)BTD(Port_Data.Data_Transfer[22],0,T30RKD.Write_Data.Output_Polarity,0,8)BTD(Port_Data.Data_Transfer[23],0,T30RKD.Write_Data.Sensor_Lockout,0,8)BTD(Port_Data.Data_Transfer[24],0,T30RKD.Write_Data.Peak_Select_Mode,0,8)BTD(Port_Data.Data_Transfer[25],0,T30RKD.Write_Data.Response_Speed,0,8)OTU(Port_Data.Port_Read.[Port])OTL(Local_Control.6);
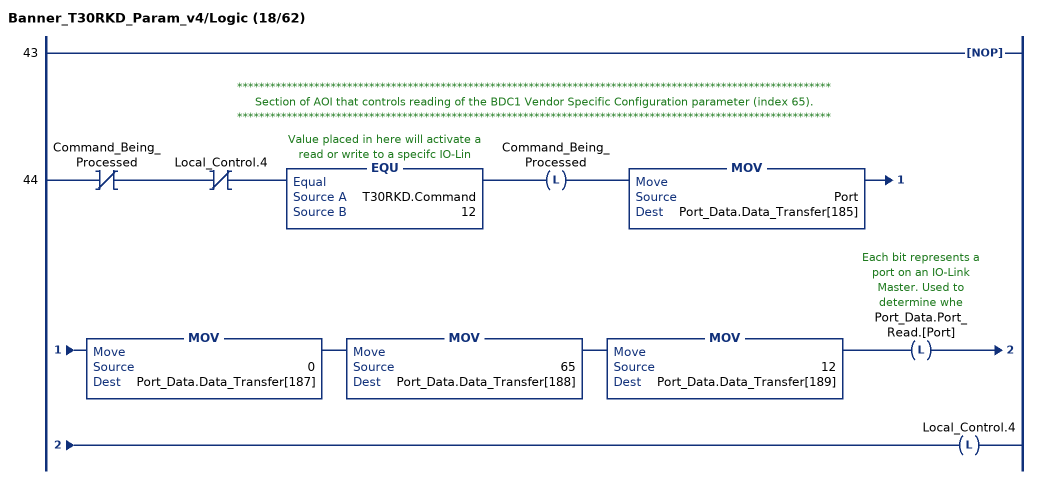
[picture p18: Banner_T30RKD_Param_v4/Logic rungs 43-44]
   43: NOP();
   // ************************************************************************************************************
   // Section of AOI that controls reading of the BDC1 Vendor Specific Configuration parameter (index 65).
   // ************************************************************************************************************
   44: XIO(Command_Being_Processed)XIO(Local_Control.4)EQU(T30RKD.Command,12)OTL(Command_Being_Processed)MOV(Port,Port_Data.Data_Transfer[185])MOV(0,Port_Data.Data_Transfer[187])MOV(65,Port_Data.Data_Transfer[188])MOV(12,Port_Data.Data_Transfer[189])OTL(Port_Data.Port_Read.[Port])OTL(Local_Control.4);
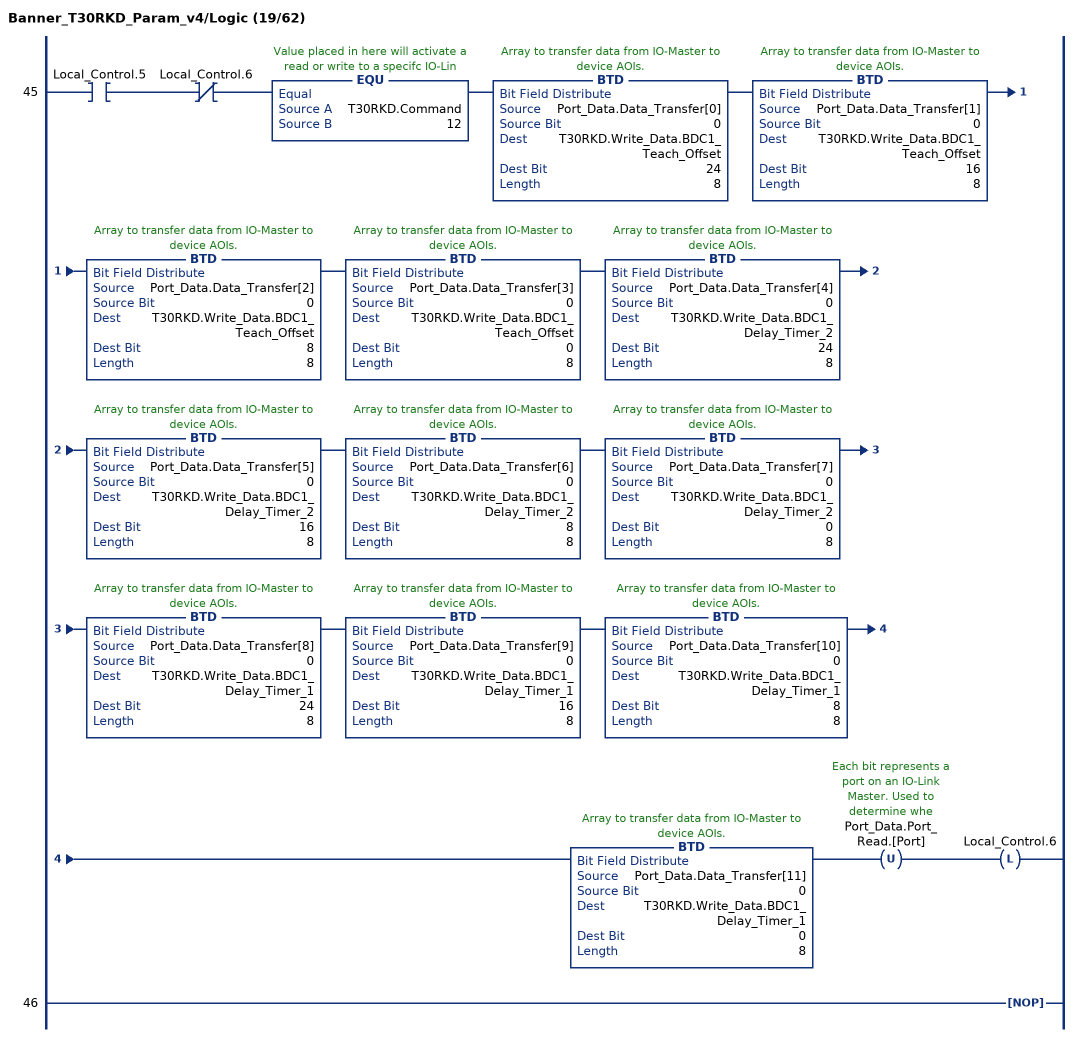
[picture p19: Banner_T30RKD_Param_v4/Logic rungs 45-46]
   45: XIC(Local_Control.5)XIO(Local_Control.6)EQU(T30RKD.Command,12)BTD(Port_Data.Data_Transfer[0],0,T30RKD.Write_Data.BDC1_Teach_Offset,24,8)BTD(Port_Data.Data_Transfer[1],0,T30RKD.Write_Data.BDC1_Teach_Offset,16,8)BTD(Port_Data.Data_Transfer[2],0,T30RKD.Write_Data.BDC1_Teach_Offset,8,8)BTD(Port_Data.Data_Transfer[3],0,T30RKD.Write_Data.BDC1_Teach_Offset,0,8)BTD(Port_Data.Data_Transfer[4],0,T30RKD.Write_Data.BDC1_Delay_Timer_2,24,8)BTD(Port_Data.Data_Transfer[5],0,T30RKD.Write_Data.BDC1_Delay_Timer_2,16,8)BTD(Port_Data.Data_Transfer[6],0,T30RKD.Write_Data.BDC1_Delay_Timer_2,8,8)BTD(Port_Data.Data_Transfer[7],0,T30RKD.Write_Data.BDC1_Delay_Timer_2,0,8)BTD(Port_Data.Data_Transfer[8],0,T30RKD.Write_Data.BDC1_Delay_Timer_1,24,8)BTD(Port_Data.Data_Transfer[9],0,T30RKD.Write_Data.BDC1_Delay_Timer_1,16,8)BTD(Port_Data.Data_Transfer[10],0,T30RKD.Write_Data.BDC1_Delay_Timer_1,8,8)BTD(Port_Data.Data_Transfer[11],0,T30RKD.Write_Data.BDC1_Delay_Timer_1,0,8)OTU(Port_Data.Port_Read.[Port])OTL(Local_Control.6);
   46: NOP();
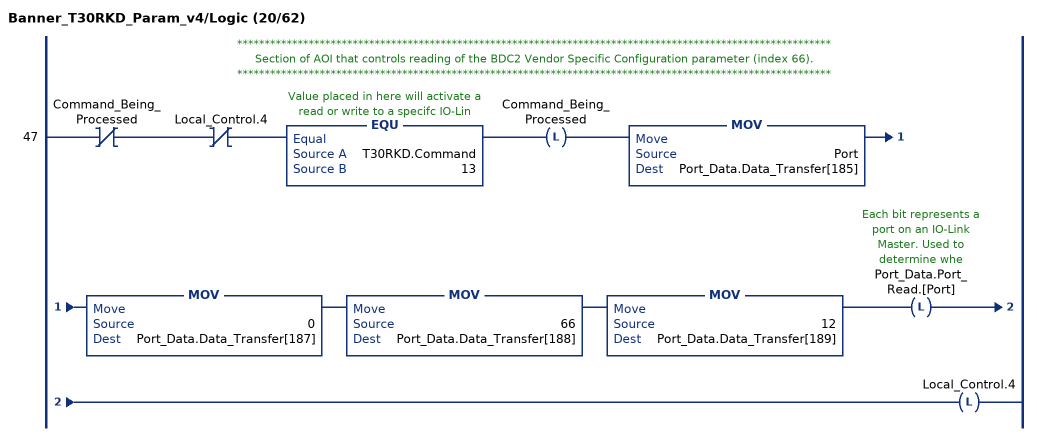
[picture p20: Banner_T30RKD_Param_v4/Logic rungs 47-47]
   // ************************************************************************************************************
   // Section of AOI that controls reading of the BDC2 Vendor Specific Configuration parameter (index 66).
   // ************************************************************************************************************
   47: XIO(Command_Being_Processed)XIO(Local_Control.4)EQU(T30RKD.Command,13)OTL(Command_Being_Processed)MOV(Port,Port_Data.Data_Transfer[185])MOV(0,Port_Data.Data_Transfer[187])MOV(66,Port_Data.Data_Transfer[188])MOV(12,Port_Data.Data_Transfer[189])OTL(Port_Data.Port_Read.[Port])OTL(Local_Control.4);
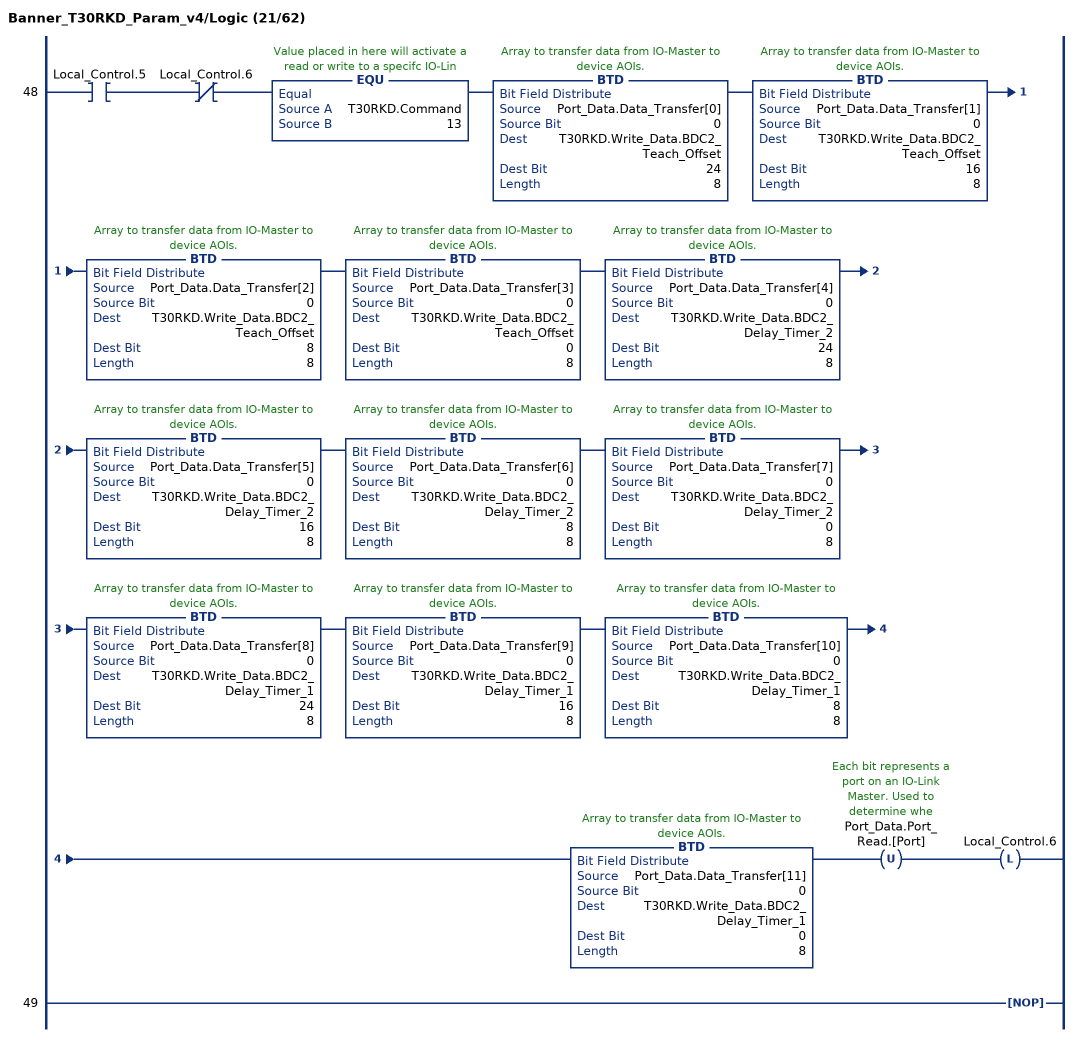
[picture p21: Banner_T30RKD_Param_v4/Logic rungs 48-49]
   48: XIC(Local_Control.5)XIO(Local_Control.6)EQU(T30RKD.Command,13)BTD(Port_Data.Data_Transfer[0],0,T30RKD.Write_Data.BDC2_Teach_Offset,24,8)BTD(Port_Data.Data_Transfer[1],0,T30RKD.Write_Data.BDC2_Teach_Offset,16,8)BTD(Port_Data.Data_Transfer[2],0,T30RKD.Write_Data.BDC2_Teach_Offset,8,8)BTD(Port_Data.Data_Transfer[3],0,T30RKD.Write_Data.BDC2_Teach_Offset,0,8)BTD(Port_Data.Data_Transfer[4],0,T30RKD.Write_Data.BDC2_Delay_Timer_2,24,8)BTD(Port_Data.Data_Transfer[5],0,T30RKD.Write_Data.BDC2_Delay_Timer_2,16,8)BTD(Port_Data.Data_Transfer[6],0,T30RKD.Write_Data.BDC2_Delay_Timer_2,8,8)BTD(Port_Data.Data_Transfer[7],0,T30RKD.Write_Data.BDC2_Delay_Timer_2,0,8)BTD(Port_Data.Data_Transfer[8],0,T30RKD.Write_Data.BDC2_Delay_Timer_1,24,8)BTD(Port_Data.Data_Transfer[9],0,T30RKD.Write_Data.BDC2_Delay_Timer_1,16,8)BTD(Port_Data.Data_Transfer[10],0,T30RKD.Write_Data.BDC2_Delay_Timer_1,8,8)BTD(Port_Data.Data_Transfer[11],0,T30RKD.Write_Data.BDC2_Delay_Timer_1,0,8)OTU(Port_Data.Port_Read.[Port])OTL(Local_Control.6);
   49: NOP();
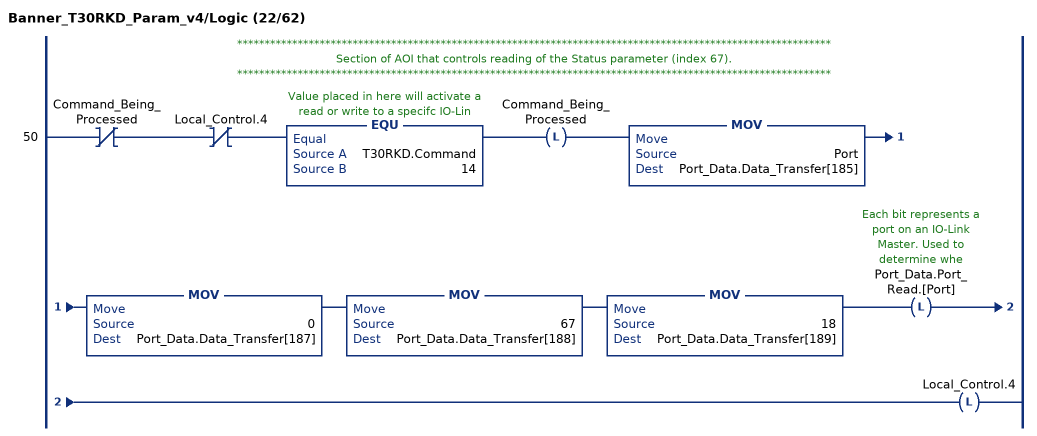
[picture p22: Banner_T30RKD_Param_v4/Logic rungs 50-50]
   // ************************************************************************************************************
   // Section of AOI that controls reading of the Status parameter (index 67).
   // ************************************************************************************************************
   50: XIO(Command_Being_Processed)XIO(Local_Control.4)EQU(T30RKD.Command,14)OTL(Command_Being_Processed)MOV(Port,Port_Data.Data_Transfer[185])MOV(0,Port_Data.Data_Transfer[187])MOV(67,Port_Data.Data_Transfer[188])MOV(18,Port_Data.Data_Transfer[189])OTL(Port_Data.Port_Read.[Port])OTL(Local_Control.4);
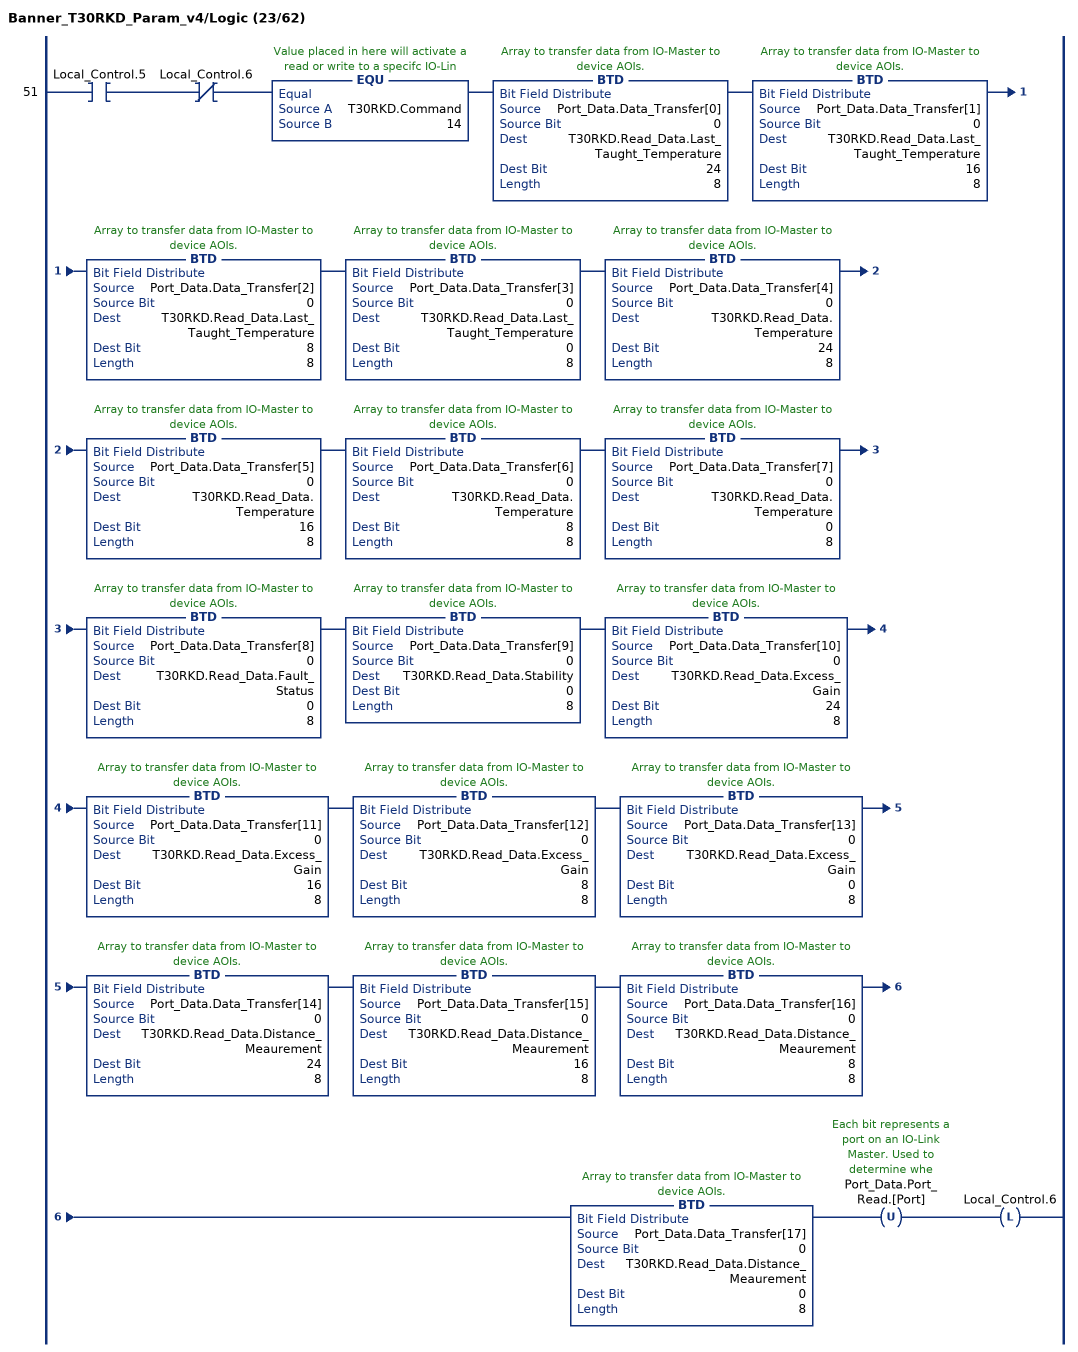
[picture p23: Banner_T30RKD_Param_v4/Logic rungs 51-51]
   51: XIC(Local_Control.5)XIO(Local_Control.6)EQU(T30RKD.Command,14)BTD(Port_Data.Data_Transfer[0],0,T30RKD.Read_Data.Last_Taught_Temperature,24,8)BTD(Port_Data.Data_Transfer[1],0,T30RKD.Read_Data.Last_Taught_Temperature,16,8)BTD(Port_Data.Data_Transfer[2],0,T30RKD.Read_Data.Last_Taught_Temperature,8,8)BTD(Port_Data.Data_Transfer[3],0,T30RKD.Read_Data.Last_Taught_Temperature,0,8)BTD(Port_Data.Data_Transfer[4],0,T30RKD.Read_Data.Temperature,24,8)BTD(Port_Data.Data_Transfer[5],0,T30RKD.Read_Data.Temperature,16,8)BTD(Port_Data.Data_Transfer[6],0,T30RKD.Read_Data.Temperature,8,8)BTD(Port_Data.Data_Transfer[7],0,T30RKD.Read_Data.Temperature,0,8)BTD(Port_Data.Data_Transfer[8],0,T30RKD.Read_Data.Fault_Status,0,8)BTD(Port_Data.Data_Transfer[9],0,T30RKD.Read_Data.Stability,0,8)BTD(Port_Data.Data_Transfer[10],0,T30RKD.Read_Data.Excess_Gain,24,8)BTD(Port_Data.Data_Transfer[11],0,T30RKD.Read_Data.Excess_Gain,16,8)BTD(Port_Data.Data_Transfer[12],0,T30RKD.Read_Data.Excess_Gain,8,8)BTD(Port_Data.Data_Transfer[13],0,T30RKD.Read_Data.Excess_Gain,0,8)BTD(Port_Data.Data_Transfer[14],0,T30RKD.Read_Data.Distance_Meaurement,24,8)BTD(Port_Data.Data_Transfer[15],0,T30RKD.Read_Data.Distance_Meaurement,16,8)BTD(Port_Data.Data_Transfer[16],0,T30RKD.Read_Data.Distance_Meaurement,8,8)BTD(Port_Data.Data_Transfer[17],0,T30RKD.Read_Data.Distance_Meaurement,0,8)OTU(Port_Data.Port_Read.[Port])OTL(Local_Control.6);
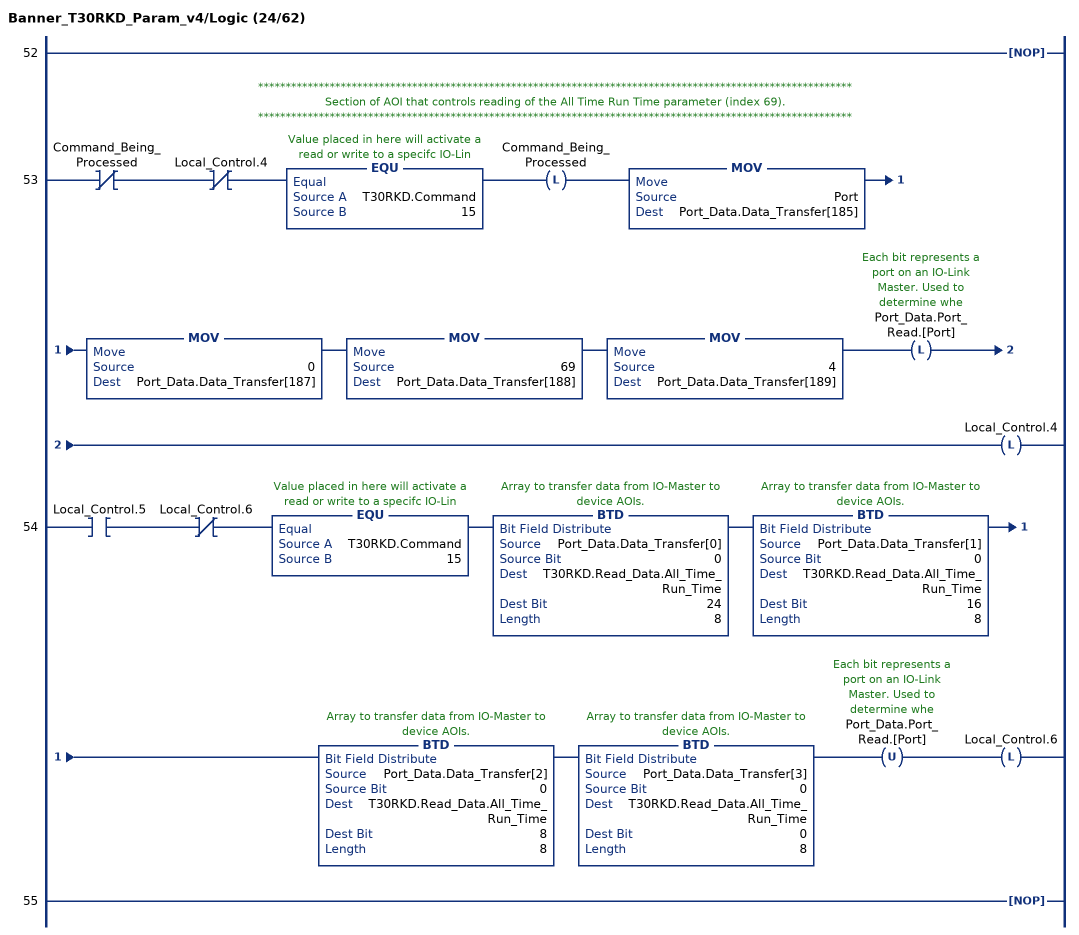
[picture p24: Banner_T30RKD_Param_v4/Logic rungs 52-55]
   52: NOP();
   // ************************************************************************************************************
   // Section of AOI that controls reading of the All Time Run Time parameter (index 69).
   // ************************************************************************************************************
   53: XIO(Command_Being_Processed)XIO(Local_Control.4)EQU(T30RKD.Command,15)OTL(Command_Being_Processed)MOV(Port,Port_Data.Data_Transfer[185])MOV(0,Port_Data.Data_Transfer[187])MOV(69,Port_Data.Data_Transfer[188])MOV(4,Port_Data.Data_Transfer[189])OTL(Port_Data.Port_Read.[Port])OTL(Local_Control.4);
   54: XIC(Local_Control.5)XIO(Local_Control.6)EQU(T30RKD.Command,15)BTD(Port_Data.Data_Transfer[0],0,T30RKD.Read_Data.All_Time_Run_Time,24,8)BTD(Port_Data.Data_Transfer[1],0,T30RKD.Read_Data.All_Time_Run_Time,16,8)BTD(Port_Data.Data_Transfer[2],0,T30RKD.Read_Data.All_Time_Run_Time,8,8)BTD(Port_Data.Data_Transfer[3],0,T30RKD.Read_Data.All_Time_Run_Time,0,8)OTU(Port_Data.Port_Read.[Port])OTL(Local_Control.6);
   55: NOP();
